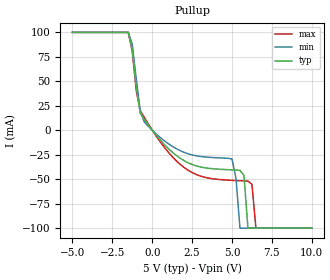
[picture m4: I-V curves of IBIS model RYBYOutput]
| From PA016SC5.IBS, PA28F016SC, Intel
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|****************Ready/Busy Output Model*****************************
[Model]   RYBYOutput
Model_type   Output
|   For RY/BY#
Vinl = 0.8V
Vinh = 2.0V
| Variable   typ   min   max
C_comp   9.61p   NA   11.6p
[Voltage Range]   5.0V   4.5V   5.5V
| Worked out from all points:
|   slope of the pullup table from 0 to 0.75 V, typ, clamps not added: 51.8 ohm
[Pulldown]
| [Pullup] and [Pulldown] IV curves include only the current through
| the channels of output driver transistors when outputs are enabled
| with OE# = VIL.  Although the output driver transistors have np and
| pn diodes inherently created by CMOS IC fabrication between the
| drain and bulk of n-channel and p-channel CMOS transistors,
| the current through these junction diodes is not included in
| [Pullup] or [Pulldown].  Instead that drain/bulk diode current is
| included in the [POWER_clamp] or [GND_clamp] sections, which are
| not dependent on the state of OE# or output data value.  The RY/BY#
| Pulldown information is not provided for this device.  The table
| below is for the compatibility with some IBIS parsers.
|Voltage   I(typ)   I(min)   I(max)
-5V       0A         0A         0A
0V        0A         0A         0A
5V        0A         0A         0A
10V       0A         0A         0A
[GND_clamp]
| The RY/BY# pin is always active and does NOT float to tri-state when
| the chip is deselected or when the data outputs are disabled.
| Therefore, the table below is included for the compatibility with
| some IBIS parsers.
|Voltage   I(typ)   I(min)   I(max)
-5V       0A         0A         0A
0V        0A         0A         0A
5V        0A         0A         0A
10V       0A         0A         0A
[Pullup]
| (Voltages for [Pullup] and [POWER_clamp] are specified with
| negative respect to Vcc.  Reference the IBIS documentation
| for more information regarding Vtable = Vcc - Voutput.
| This method keeps -Vds constant for the values in all three
| columns across a line of the table.)
| [Pullup] and [Pulldown] IV curves include only the current through
| the channels of output driver transistors when outputs are enabled
| with OE# = VIL.  Although the output driver transistors have np and
| pn diodes inherently created by CMOS IC fabrication between the
| drain and bulk of n-channel and p-channel CMOS transistors,
| the current through these junction diodes is not included in
| [Pullup] or [Pulldown].  Instead that drain/bulk diode current is
| included in the [POWER_clamp] or [GND_clamp] sections, which are
| not dependent on the state of OE# or output data value.
|Voltage  I(typ)   I(min)   I(max)
-5V       100mA      100mA      100mA
-1.5V     100mA      100mA      100mA
-750mV    17.42mA    20.09mA    20.13mA
250mV     -5.027mA   -3.811mA   -5.927mA
2.25V     -33.22mA   -24.02mA   -40.83mA
5V        -40.47mA   -29.33mA   -51.2mA
5.5V      -40.97mA   -100mA     -51.56mA
5.75V     -46.15mA   -100mA     -51.71mA
6V        -100mA     -100mA     -51.94mA
6.25V     -100mA     -100mA     -55.18mA
6.5V      -100mA     -100mA     -100mA
10V       -100mA     -100mA     -100mA
[POWER_clamp]
| The RY/BY# pin is always active and does NOT float to tri-state when
| the chip is deselected or when the data outputs are disabled.
| Therefore, the table below is included for the compatibility with
| some IBIS parsers.
|Voltage  I(typ)   I(min)   I(max)
-5V       0A         0A         0A
0V        0A         0A         0A
5V        0A         0A         0A
10V       0A         0A         0A
[Ramp]
| The RY/BY# Ramp information is not provided for this device.  The table
| below is for the compatibility with some IBIS parsers.
| Variable   typ   min   max
 dV/dt_r   0V/0ns   0V/0ns   0V/0ns
 dV/dt_f   0V/0ns   0V/0ns   0V/0ns
